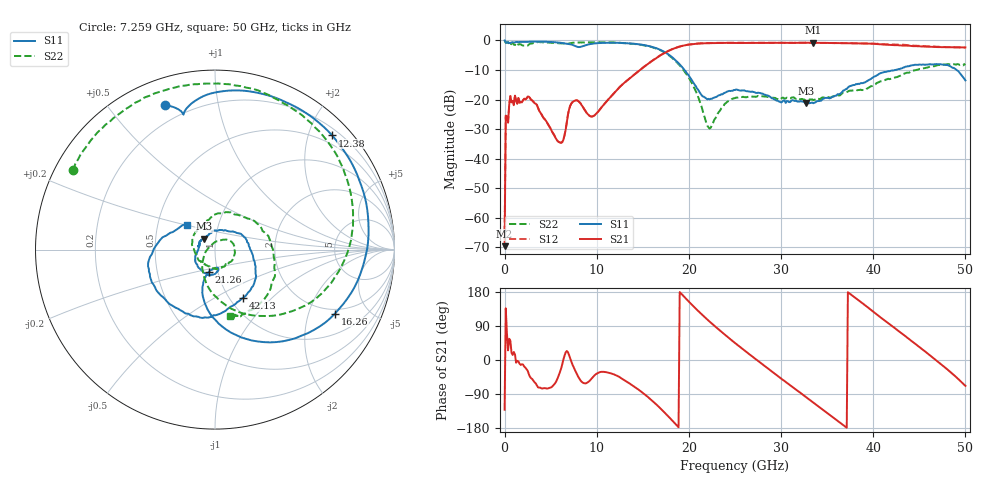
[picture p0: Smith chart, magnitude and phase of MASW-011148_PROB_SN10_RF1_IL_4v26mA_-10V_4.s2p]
!Keysight Technologies,N5247A,US51170177,A.10.64.09
!Date: Saturday, May 29, 2021 13:32:21
!Correction: S11(Full 2 Port(1,2))
!S21(Full 2 Port(1,2))
!S12(Full 2 Port(1,2))
!S22(Full 2 Port(1,2))
!S2P File: Measurements: S11, S21, S12, S22:
# Hz S  dB  R 50
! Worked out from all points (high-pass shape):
!   401 points, 10 MHz to 50 GHz, reference 50 ohm
!   highest |S21| = -0.79 dB at 33.5 GHz (marker M1); lowest = -69.6 dB at 10 MHz (marker M2)
!   |S21| within 3 dB of the highest: 17.64 GHz to end of sweep
!   lowest |S11| = -21.3 dB at 32.75 GHz (marker M3), VSWR 1.19, Z = 44 + j5.47 ohm
!   |S11| at or under -10 dB: 19.52 GHz to 42.37 GHz (22.85 GHz wide, 73.9 % of centre); 49.06 GHz to end of sweep
!   |S22| runs from -29.8 to 0.0 dB; largest |S21 - S12| = 0.031
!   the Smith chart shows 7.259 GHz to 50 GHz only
!   S11 on the Smith chart (normalised r, x): 7.259 GHz: 0.12, +0.70; 12.38 GHz: 0.32, +2.42; 16.26 GHz: 1.80, -3.01; 21.26 GHz: 0.91, -0.23; 42.13 GHz: 1.15, -0.68; 50 GHz: 0.70, +0.20
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1e7  -0.01 -1.8  -69.59 -131.3  -65.03 -135.9  -0.02 -1.0
3.84925e8  -0.66 -52.0  -27.77 25.5  -27.76 25.5  -0.51 -27.1
2.25955e9  -0.52 -160.5  -19.97 -20.0  -19.93 -20.0  -1.76 -105.2
6.0088e9  -0.76 127.0  -34.52 -32.3  -34.49 -32.4  -0.97 167.8
7.25855e9  -1.40 109.2  -21.32 -4.9  -21.29 -4.9  -0.87 150.8
8.383325e9  -2.06 102.4  -21.96 -57.8  -21.93 -57.8  -0.70 133.2
1.238252e10  -0.80 44.2  -16.14 -43.7  -16.14 -43.7  -0.77 73.0
1.625675e10  -2.41 -28.1  -6.40 -112.6  -6.35 -112.5  -2.52 1.3
1.675665e10  -2.99 -39.3  -5.36 -124.0  -5.31 -123.9  -3.11 -10.1
1.913118e10  -8.53 -92.3  -1.98 176.1  -1.93 176.1  -8.90 -71.3
2.125575e10  -17.91 -104.9  -1.03 123.7  -0.97 123.8  -21.37 -140.6
2.225555e10  -19.94 -83.8  -0.91 101.2  -0.91 101.2  -29.82 126.9
2.5005e10  -16.77 -101.4  -0.87 44.9  -0.77 44.9  -19.49 18.3
2.837932e10  -18.56 -158.3  -0.83 -18.7  -0.79 -18.9  -19.00 -34.6
3.275345e10  -21.32 134.2  -0.79 -98.7  -0.76 -98.9  -20.01 -111.0
3.337832e10  -20.99 120.3  -0.80 -110.3  -0.80 -110.5  -19.93 -125.7
3.35033e10  -21.24 117.2  -0.79 -112.6  -0.80 -112.7  -20.17 -126.2
3.75025e10  -15.44 31.3  -0.96 174.3  -0.95 174.7  -16.97 152.0
4.175165e10  -10.41 -52.0  -1.50 94.8  -1.33 95.6  -13.12 64.1
4.212658e10  -10.17 -59.8  -1.56 88.2  -1.34 88.6  -12.80 58.3
4.625075e10  -8.09 -133.0  -2.14 10.4  -2.04 9.7  -8.74 -24.2
5e10  -13.51 138.8  -2.37 -68.3  -2.41 -69.1  -8.36 -77.2
